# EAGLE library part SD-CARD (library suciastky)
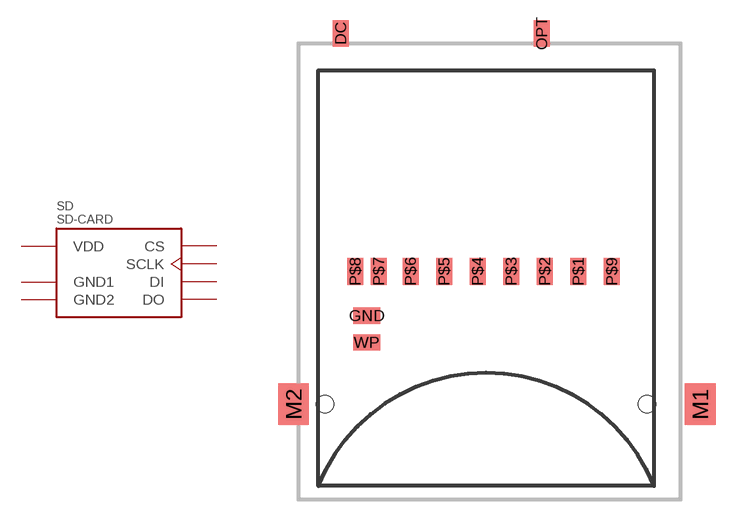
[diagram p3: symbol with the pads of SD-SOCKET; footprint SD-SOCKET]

Designator prefix SD

## SD-CARD  [SD-SOCKET]
DC  GND1  pwr
GND  GND1  pwr
M1  GND1  pwr
M2  GND1  pwr
OPT  GND1  pwr
P$1  CS  in
P$2  DI  in
P$3  GND1  pwr
P$4  VDD
P$5  SCLK  in
P$6  GND2  pwr
P$7  DO  out
WP  GND1  pwr

## Footprint SD-SOCKET (pad centres in mm)
smd 1.2 x 2: DC -10.83,17.75; OPT 4.15,17.75; P$1 6.87,0; P$2 4.37,0; P$3 1.87,0; P$4 -0.63,0; P$5 -3.13,0; P$6 -5.63,0; P$7 -8,0; P$8 -9.75,0; P$9 9.37,0
smd 2 x 1.2: GND -8.9,-3.3; WP -8.9,-5.3
smd 2.3 x 3.1: M1 15.95,-9.9; M2 -14.35,-9.9
hole 1.3 at 12,-9.9
hole 1.3 at -12,-9.9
